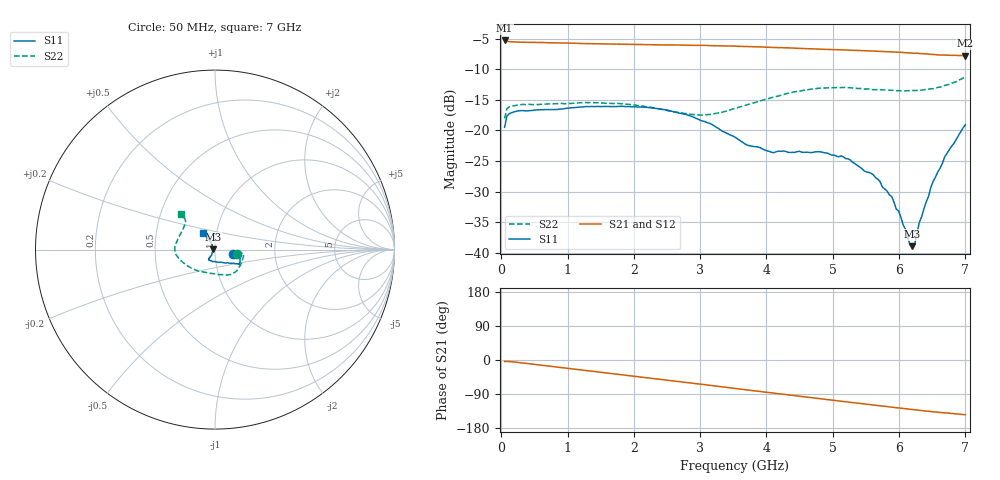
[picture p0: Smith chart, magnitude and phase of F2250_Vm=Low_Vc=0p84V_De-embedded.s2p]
! Integrated Device Technology
! Corporate Headquarters
! 6024 Silver Creek Valley Road
! San Jose, CA 95138  USA
! Phone:  1-408-284-8200
! Toll Free:  1-800-223-1366
! Webpage:  http://www.idt.com/
! Timing and RF Division
! 515 Groton Road, Suite 102
! Westford, MA 01886-6024
! Device:  F2250
! Description: Voltage Variable RF Attenuator
! Frequency:  50.0 -  6000.00 MHz
! Package:  3x3 mm Thin QFN Plastic Package: 16 pin
! Ports:  2 RF, 3 DC
!  Pin  1  = GND
!  Pin  2  = NC
!  Pin  3  = RF1  = Port 1
!  Pin  4  = NC
!  Pin  5  = GND
!  Pin  6  = GND
!  Pin  7  = GND
!  Pin  8  = GND
!  Pin  9  = NC
!  Pin 10  = RF2  = Port 2
!  Pin 11  = NC
!  Pin 12  = GND
!  Pin 13  = GND
!  Pin 14  = VCNTRL
!  Pin 15  = VDD
!  Pin 16  = VMODE
! Vcntrl:  0.840 Volts
! Vmode:  +0.000 Volts
! Vdd:  +3.30  Volts
! Current:  1.172 mA
! Data:  The device was measured on a the F2250 evaluation board which has
!  individual transmission lines to the RF pins.  Data was collected
!  using a calibrated network analyzer.  The evaluation board was
!  de-embedded using a TRL calibration technique.
!  The reference plane is the edge of the package pin.
! Misc:  SN 10
!  Action Tracker AT0258
! Date Measured:  2014-11-26
! Date:  2015-10-15  MJV
! Note:
!  Integrated Device Technology supplies this data as a sample of measured
!  data at the package pin for this product.  Your particular data for this
!  product may vary.
!  Data was taken at 25 degrees C.
!  Integrated Device Technology reserves the right to change this data at anytime.
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# GHz S dB R 50
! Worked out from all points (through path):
!   201 points, 50 MHz to 7 GHz, reference 50 ohm
!   highest |S21| = -5.29 dB at 50 MHz (marker M1); lowest = -7.8 dB at 7 GHz (marker M2)
!   group delay of S21, straight-line fit = 57.9 ps
!   lowest |S11| = -38.9 dB at 6.201 GHz (marker M3), VSWR 1.02, Z = 48.9 + j0.0545 ohm
!   |S11| at or under -10 dB: start of sweep to end of sweep
!   |S22| runs from -18.0 to -11.3 dB; largest |S21 - S12| = 0.0017
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0.05  -19.48 -13.9  -5.29 -4.0  -5.28 -4.0  -18.04 -12.1
0.08475  -17.63 -7.7  -5.43 -3.7  -5.44 -3.7  -16.44 -7.6
0.22375  -16.86 -7.3  -5.54 -5.9  -5.55 -5.9  -15.90 -9.9
1.2315  -16.15 -26.3  -5.80 -27.0  -5.79 -27.0  -15.45 -42.7
2.37825  -16.45 -32.1  -6.02 -50.5  -6.01 -50.5  -16.45 -70.0
3.0385  -18.46 -39.6  -6.11 -64.5  -6.10 -64.5  -17.47 -100.5
3.525  -21.09 -56.6  -6.22 -75.0  -6.23 -75.0  -16.39 -128.9
3.69875  -22.34 -66.3  -6.29 -78.8  -6.29 -78.8  -15.83 -137.5
4.081  -23.58 -91.1  -6.42 -87.0  -6.43 -87.0  -14.64 -154.3
4.7065  -23.55 -119.9  -6.67 -100.2  -6.66 -100.2  -13.23 -172.5
5.2625  -24.80 -123.4  -6.91 -111.6  -6.90 -111.7  -13.02 174.8
5.61  -27.23 -122.5  -7.02 -118.8  -7.04 -118.8  -13.34 166.4
5.85325  -30.52 -124.6  -7.14 -123.7  -7.15 -123.7  -13.43 160.0
5.888  -30.78 -125.8  -7.16 -124.4  -7.16 -124.4  -13.43 159.4
5.99225  -33.15 -134.2  -7.21 -126.6  -7.21 -126.6  -13.49 155.9
6.166  -38.70 -163.7  -7.32 -130.0  -7.33 -130.0  -13.50 150.1
6.20075  -38.89 177.2  -7.37 -130.7  -7.35 -130.8  -13.47 148.9
6.2355  -38.61 159.9  -7.38 -131.4  -7.37 -131.4  -13.48 147.7
6.305  -35.00 139.8  -7.42 -132.8  -7.43 -132.8  -13.41 145.4
6.5135  -28.32 119.8  -7.59 -136.5  -7.59 -136.6  -13.17 139.0
6.68725  -24.32 118.6  -7.69 -139.5  -7.68 -139.5  -12.64 135.0
7  -19.07 126.1  -7.78 -144.5  -7.79 -144.5  -11.27 133.1
